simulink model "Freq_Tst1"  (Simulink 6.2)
settings: Solver=ode45  StartTime=0.0  StopTime=400  FixedStep=0.0005  MaxStep=0.002  RelTol=1e-3
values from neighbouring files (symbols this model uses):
  r2d = 180/pi    (= 57.2957795131)    [Pl.m]    (also in run.m)
undefined symbols (not defined in the file or in its folder): Ar, Br, Cr, Dr, KJmix, KSmix

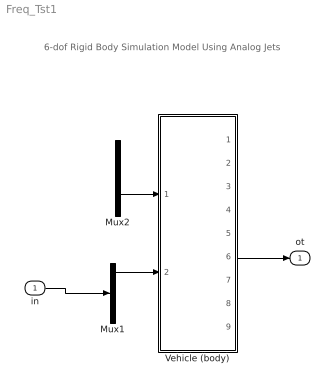
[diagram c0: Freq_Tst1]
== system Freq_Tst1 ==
  note: 6-dof Rigid Body Simulation Model Using Analog Jets
  in : Inport  Port=1  LatchInput=off
  Mux1 : Mux  Inputs=3
  Mux2 : Mux
  Vehicle (body) : Subsystem
  ot : Outport
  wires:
  Mux2/1 -> Vehicle (body)/1(Jet_PQR_Nz)
  Mux1/1 -> Vehicle (body)/2(Aer_pqr)
  in/1 -> Mux1/2
  Vehicle (body)/6(q) -> ot/1

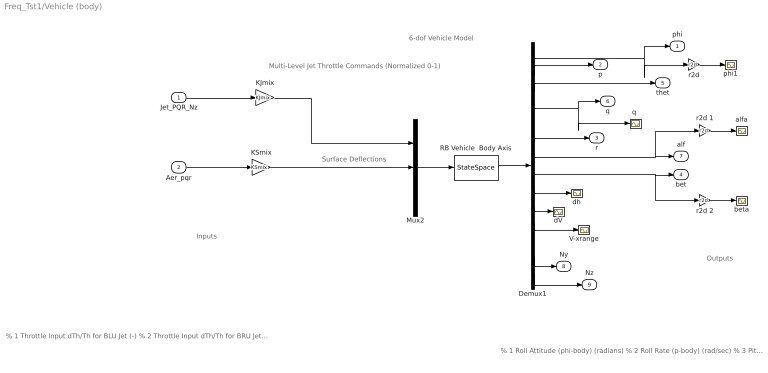
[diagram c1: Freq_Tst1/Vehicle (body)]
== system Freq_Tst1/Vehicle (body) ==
  note: Surface Deflections
  note: Multi-Level Jet Throttle Commands (Normalized 0-1)
  note: % 1 Roll Attitude (phi-body) (radians) % 2 Roll Rate (p-body) (rad/sec) % 3 Pitch Attitude (thet-bdy) (radians) % 4 Pitch Rate (q-body) (rad/sec) % 5 Yaw Attitude (psi-body) (radians) % 6 Yaw Rate (r-body) (rad/sec) % 7 Angle of attack, alfa, (radians) % 8 Angle of sideslip, beta, (radian) % 9 Change in Altitude, delta-h, (feet) % 10 Forward Acceleration (V-dot) (ft/sec) % 11 Cross Range Velocity (Vcr) (ft/sec) % 12 CG Acceleration along X axis, (ft/sec^2) % 13 CG Acceleration along Y axis, (ft/sec^2) % 14 CG Acceleration along Z axis, (ft/sec^2)
  note: % 1 Throttle Input dTh/Th for BLU Jet (-) % 2 Throttle Input dTh/Th for BRU Jet (-) % 3 Throttle Input dTh/Th for BLD Jet (-) % 4 Throttle Input dTh/Th for BRD Jet (-) % 5 Throttle Input dTh/Th for BL+Y Jet (-) % 6 Throttle Input dTh/Th for BR-Y Jet (-) % 7 Throttle Input dTh/Th for FU Jet (-) % 8 Throttle Input dTh/Th for FD Jet (-) % 9 Throttle Input dTh/Th for FL Jet (-) % 10 Throttle Input dTh/Th for FR Jet (-) % 11 Left Outbrd Elevon Deflection (radians) % 12 Left Inboard Elevon Deflection (radians) % 13 Right Inbrd Elevon Deflection (radians) % 14 Right Outbrd Elevon Deflection (radians) % 15 Vertical Rudder Deflection (radians) % 16 Gust Veloc, Azim-Elev Angles=(45,90) (deg)
  note: 6-dof Vehicle Model
  note: Inputs
  note: Outputs
  Jet_PQR_Nz : Inport  Port=1  LatchInput=off
  Aer_pqr : Inport  Port=2  LatchInput=off
  Demux1 : Demux  Outputs=14
  KJmix : Gain  Gain=KJmix  Multiplication=Matrix(K*u)
  KSmix : Gain  Gain=KSmix  Multiplication=Matrix(K*u)
  Mux2 : Mux  Inputs=[11, 5, 1]
  RB Vehicle  Body Axis : StateSpace  A=Ar  B=Br  C=Cr  D=Dr
  V-xrange : Scope
  alfa : Scope
  beta : Scope
  dV : Scope
  dh : Scope
  phi1 : Scope
  "q " : Scope
  r2d : Gain  Gain=r2d
  r2d 1 : Gain  Gain=r2d
  r2d 2 : Gain  Gain=r2d
  phi : Outport
  p : Outport  Port=2
  r : Outport  Port=3
  bet : Outport  Port=4
  thet : Outport  Port=5
  q : Outport  Port=6
  alf : Outport  Port=7
  Ny : Outport  Port=8
  Nz : Outport  Port=9
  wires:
  Mux2/1 -> RB Vehicle  Body Axis/1
  KSmix/1 -> Mux2/2
  Demux1/2 -> p/1
  Demux1/4 -> q/1, "q "/1
  Demux1/6 -> r/1
  Demux1/7 -> alf/1, r2d 1/1
  Demux1/8 -> bet/1, r2d 2/1
  Aer_pqr/1 -> KSmix/1
  Demux1/3 -> thet/1
  Demux1/1 -> phi/1, r2d/1
  RB Vehicle  Body Axis/1 -> Demux1/1
  Demux1/9 -> dh/1
  Demux1/10 -> dV/1
  Demux1/14 -> Nz/1
  r2d 1/1 -> alfa/1
  r2d 2/1 -> beta/1
  Demux1/13 -> Ny/1
  Demux1/11 -> V-xrange/1
  r2d/1 -> phi1/1
  Jet_PQR_Nz/1 -> KJmix/1
  KJmix/1 -> Mux2/1
